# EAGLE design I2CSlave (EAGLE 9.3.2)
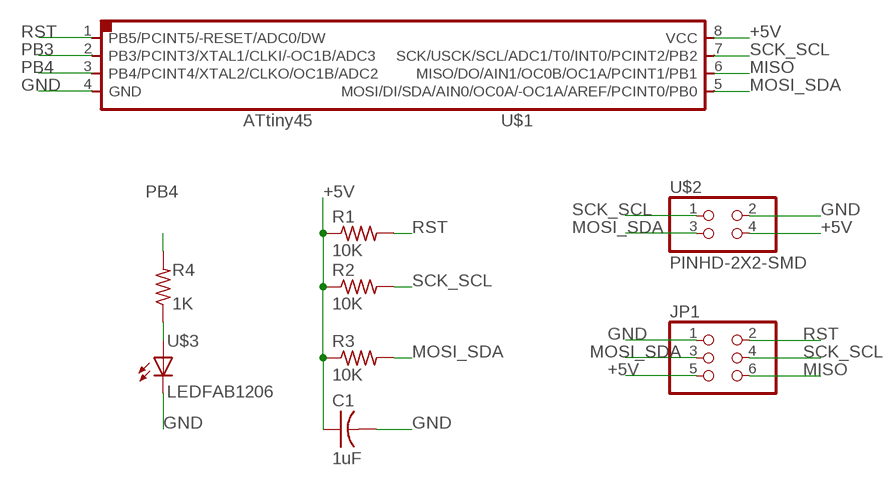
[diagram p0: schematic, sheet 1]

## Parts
C1  1uF  CAP-US1206FAB  [C1206FAB]
JP1  PINHD-2X3-SMD  [2X03SMD]
R1  10K  RES-US1206FAB  [R1206FAB]
R2  10K  RES-US1206FAB  [R1206FAB]
R3  10K  RES-US1206FAB  [R1206FAB]
R4  1K  RES-US1206FAB  [R1206FAB]
U$1  ATTINY45SI  [SOIC8]
U$2  PINHD-2X2-SMD  [2X02SMD]
U$3  LEDFAB1206  [LED1206FAB]

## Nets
+5V: C1.1 JP1.5 R1.1 R2.1 R3.1 U$1.8(VCC) U$2.4
GND: C1.2 JP1.1 U$1.4(GND) U$2.2 U$3.2(C)
MISO: JP1.6 U$1.6(MISO/DO/AIN1/OC0B/OC1A/PCINT1/PB1)
MOSI_SDA: JP1.3 R3.2 U$1.5(MOSI/DI/SDA/AIN0/OC0A/-OC1A/AREF/PCINT0/PB0) U$2.3
N$1: R4.1 U$3.1(A)
PB3: U$1.2(PB3/PCINT3/XTAL1/CLKI/-OC1B/ADC3)
PB4: R4.2 U$1.3(PB4/PCINT4/XTAL2/CLKO/OC1B/ADC2)
RST: JP1.2 R1.2 U$1.1(PB5/PCINT5/-RESET/ADC0/DW)
SCK_SCL: JP1.4 R2.2 U$1.7(SCK/USCK/SCL/ADC1/T0/INT0/PCINT2/PB2) U$2.1

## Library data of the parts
C1 = fab:CAP-US
JP1 = fab:PINHD-2X3-SMD: PIN HEADER
R1-R4 = fab:RES-US: Resistor (US Symbol)
U$1 = fab:ATTINY45
U$2 = fab:PINHD-2X2-SMD
U$3 = fab:LED: LED

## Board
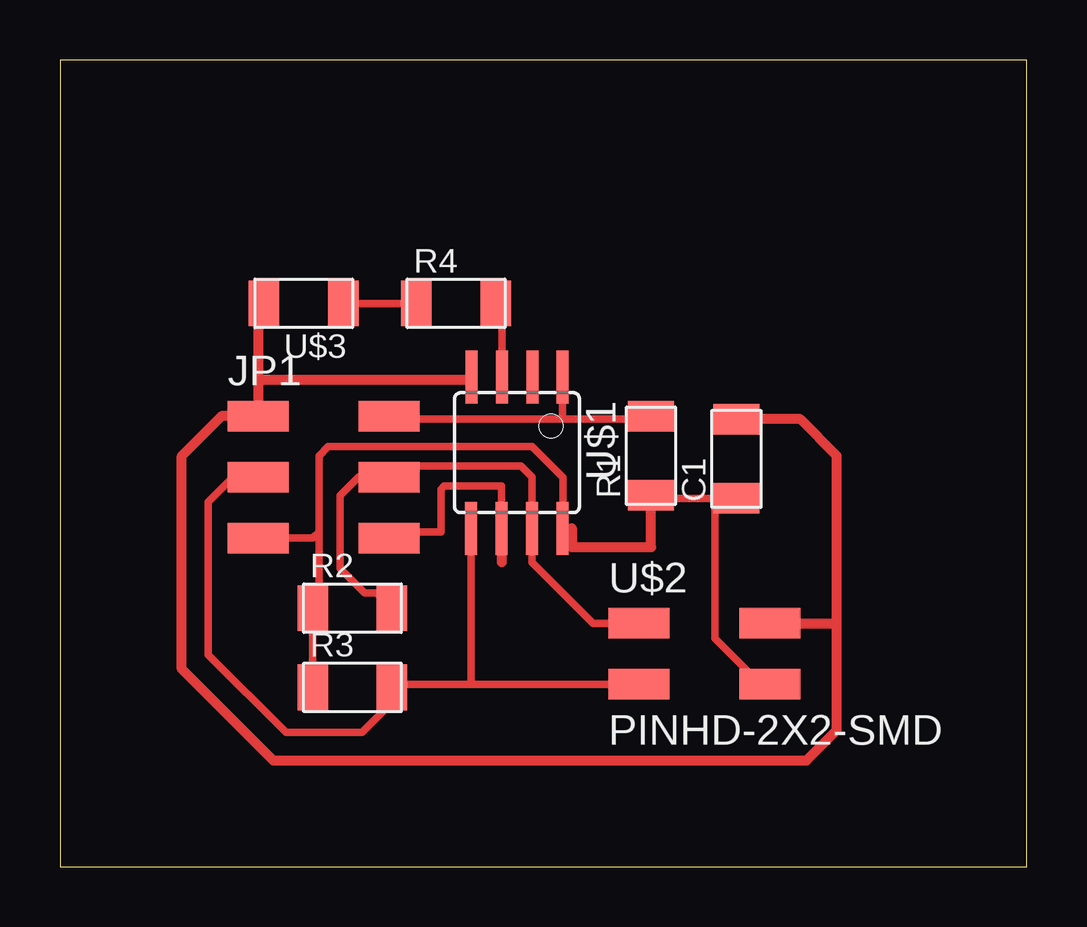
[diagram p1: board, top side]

Size 40.31 x 33.65 mm. Coordinates in mm from the lower left corner, seen from the top.
Outline: 0,0 40.31,0 40.31,33.65 0,33.65 0,0
Copper layers (1*16): Top 0.035mm / dielectric 1.5mm / Bottom 0.035mm
Design rules "default *": minimum track width 6mil, minimum drill 0.35mm, track to track 0.46mm, track to pad 0.46mm, pad to pad 0.46mm, via to via 0.46mm, smd to smd 0.46mm, copper to edge 0.4mm, drill to drill 6mil, minimum pad ring 10mil, minimum via ring 8mil, stop-mask expansion 4mil, vias tented up to drill 0mil, thermal gap 10mil

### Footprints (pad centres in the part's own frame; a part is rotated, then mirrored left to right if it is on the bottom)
C1206FAB = smd 1.27 x 1.905: 1 -1.651,0; 2 1.651,0
2X03SMD = smd 2.54 x 1.27: 1 -2.54,2.54; 2 2.92,2.54; 3 -2.54,0; 4 2.92,0; 5 -2.54,-2.54; 6 2.92,-2.54
R1206FAB = smd 1.27 x 1.905: 1 -1.651,0; 2 1.651,0
SOIC8 = smd 0.5 x 2.2: 1 -1.905,-3.154; 2 -0.645,-3.154; 3 0.625,-3.154; 4 1.895,-3.154; 5 1.905,3.154; 6 0.635,3.154; 7 -0.635,3.154; 8 -1.905,3.154
2X02SMD = smd 2.54 x 1.27: 1 -2.54,1.27; 2 2.92,1.27; 3 -2.54,-1.27; 4 2.92,-1.27
LED1206FAB = smd 1.27 x 1.905: 1 -1.651,0; 2 1.651,0

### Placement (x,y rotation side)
C1  28.19,17.02 90 top
JP1  10.79,16.26 0 top
R1  24.64,17.14 90 top
R2  12.19,10.79 0 top
R3  12.19,7.49 0 top
R4  16.51,23.5 0 top
U$1  19.05,17.27 180 top
U$2  26.67,8.89 0 top
U$3  10.16,23.5 180 top

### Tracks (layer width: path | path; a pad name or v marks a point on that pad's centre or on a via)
+5V
  Top 0.305: C1.1 27.3,15.37 | 27.3,15.37 24.77,15.37 R1.1 | U$2.4 29.21,7.62 27.3,9.53 27.3,15.37 | 20.98,14.1 U$1.8 | 10.79,13.97 10.79,17.14 11.18,17.53 19.68,17.53 20.98,16.23 20.98,14.1 | 20.98,14.1 20.98,13.97 | JP1.5 10.54,13.72 10.79,13.97 | 10.79,13.97 10.79,11.05 R2.1 R3.1
  Top 0.406: 20.98,13.97 20.98,14.12 U$1.8 21.34,14.12 21.34,13.34 24.64,13.34 R1.1
GND
  Top 0.406: U$3.2 8.26,23.24 8.26,20.32 | 8.26,20.32 JP1.1 6.73,18.8 5.08,17.14 5.08,8.26 8.89,4.45 31.11,4.45 32.38,5.71 32.38,10.16 | C1.2 30.86,18.67 32.38,17.14 32.38,10.16 | U$2.2 32.38,10.16 | 8.26,20.32 17.05,20.32 U$1.4
MISO
  Top 0.305: JP1.6 13.97,13.97 15.88,13.97 15.88,15.75 16,15.88 18.41,15.88 U$1.6
  Top 0.406: U$1.6 18.41,12.7
MOSI_SDA
  Top 0.305: 17.14,7.62 13.97,7.62 R3.2 13.84,6.86 12.59,5.61 9.42,5.61 6.18,8.85 6.18,15.21 7.22,16.26 JP1.3 | 17.14,7.62 U$2.3 | U$1.5 17.14,7.62
N$1
  Top 0.305: R4.1 U$3.1
PB4
  Top 0.305: R4.2 18.43,23.23 U$1.3
RST
  Top 0.305: R1.2 24.51,18.8 24.38,18.67 20.95,18.67 | U$1.1 20.95,18.67 | 20.95,18.67 13.84,18.67 JP1.2
SCK_SCL
  Top 0.305: U$2.1 22.23,10.16 19.68,12.7 U$1.7 19.68,16.26 19.23,16.71 14.17,16.71 JP1.4 12.45,16.26 11.68,15.49 11.68,12.45 12.7,11.43 13.21,11.43 R2.2

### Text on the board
Reference: GND | GND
